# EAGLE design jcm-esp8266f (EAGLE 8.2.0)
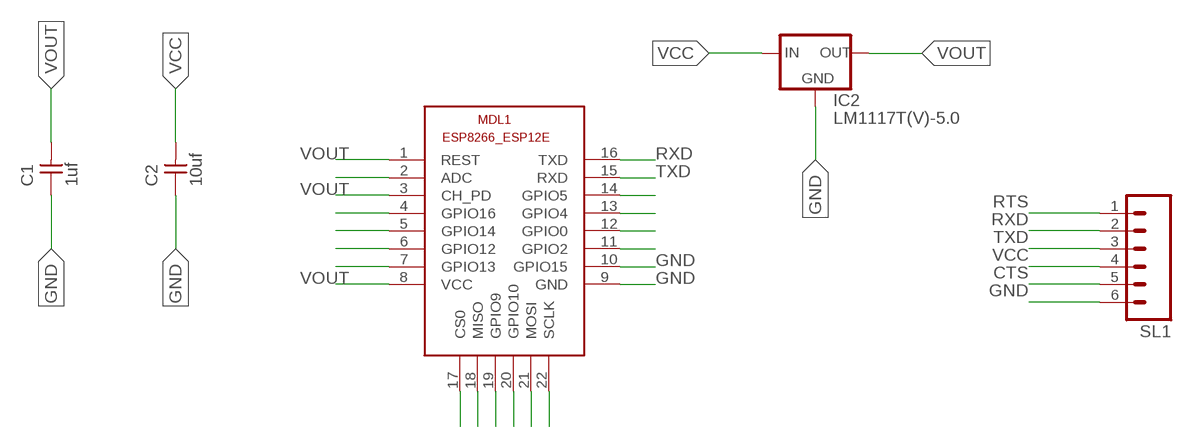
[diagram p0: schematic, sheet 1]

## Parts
C1  1uf  UNPOLARIZED_CAPACITOR1206  [1206]
C2  10uf  UNPOLARIZED_CAPACITOR1206  [1206]
IC2  LM1117T(V)-5.0  [TO220V]
MDL1  ESP8266-12EESP8266-ESP12E  [ESP8266-ESP12E]
SL1  M06  [06P]

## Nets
CTS: SL1.5
GND: C1.1 C2.1 IC2.1(GND) MDL1.9(GND) MDL1.10(GPIO15) SL1.6
N$9: MDL1.14(GPIO5)
N$10: MDL1.13(GPIO4)
N$11: MDL1.12(GPIO0)
N$12: MDL1.11(GPIO2)
N$15: MDL1.22(SCLK)
N$16: MDL1.21(MOSI)
N$17: MDL1.20(GPIO10)
N$18: MDL1.19(GPIO9)
N$19: MDL1.18(MISO)
N$20: MDL1.17(CS0)
N$22: MDL1.7(GPIO13)
N$23: MDL1.6(GPIO12)
N$24: MDL1.5(GPIO14)
N$25: MDL1.4(GPIO16)
N$27: MDL1.2(ADC)
RTS: SL1.1
RXD: MDL1.16(TXD) SL1.2
TXD: MDL1.15(RXD) SL1.3
VCC: C2.2 IC2.3(IN) SL1.4
VOUT: C1.2 IC2.2(OUT) MDL1.1(REST) MDL1.3(CH_PD) MDL1.8(VCC)

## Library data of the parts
C1 C2 = FAB_Hello:UNPOLARIZED_CAPACITOR: unpolarized_capacitor
IC2 = voltage_regulator:LM1117?-*: 800mA Low-Dropout Linear Regulator Source: http://ww1.microchip.com/downloads/en/DeviceDoc/39760d.pdf; MF: Texas Instruments; MPN: LM1117T-5.0; OC_FARNELL: 1215183; OC_NEWARK: 41K3491
MDL1 = ESP8266-ESP12E:ESP8266-12E: ESP8266-12E with additional I/O and GPIO04/05 corrected The author cannot warrant that this library is free from error or will meet your specific requirements. Created by PuceBaboon.com. Komagane, Nagano, JAPAN
SL1 = con-amp-quick:M06: AMP QUICK CONNECTOR; OC_FARNELL: unknown; OC_NEWARK: unknown

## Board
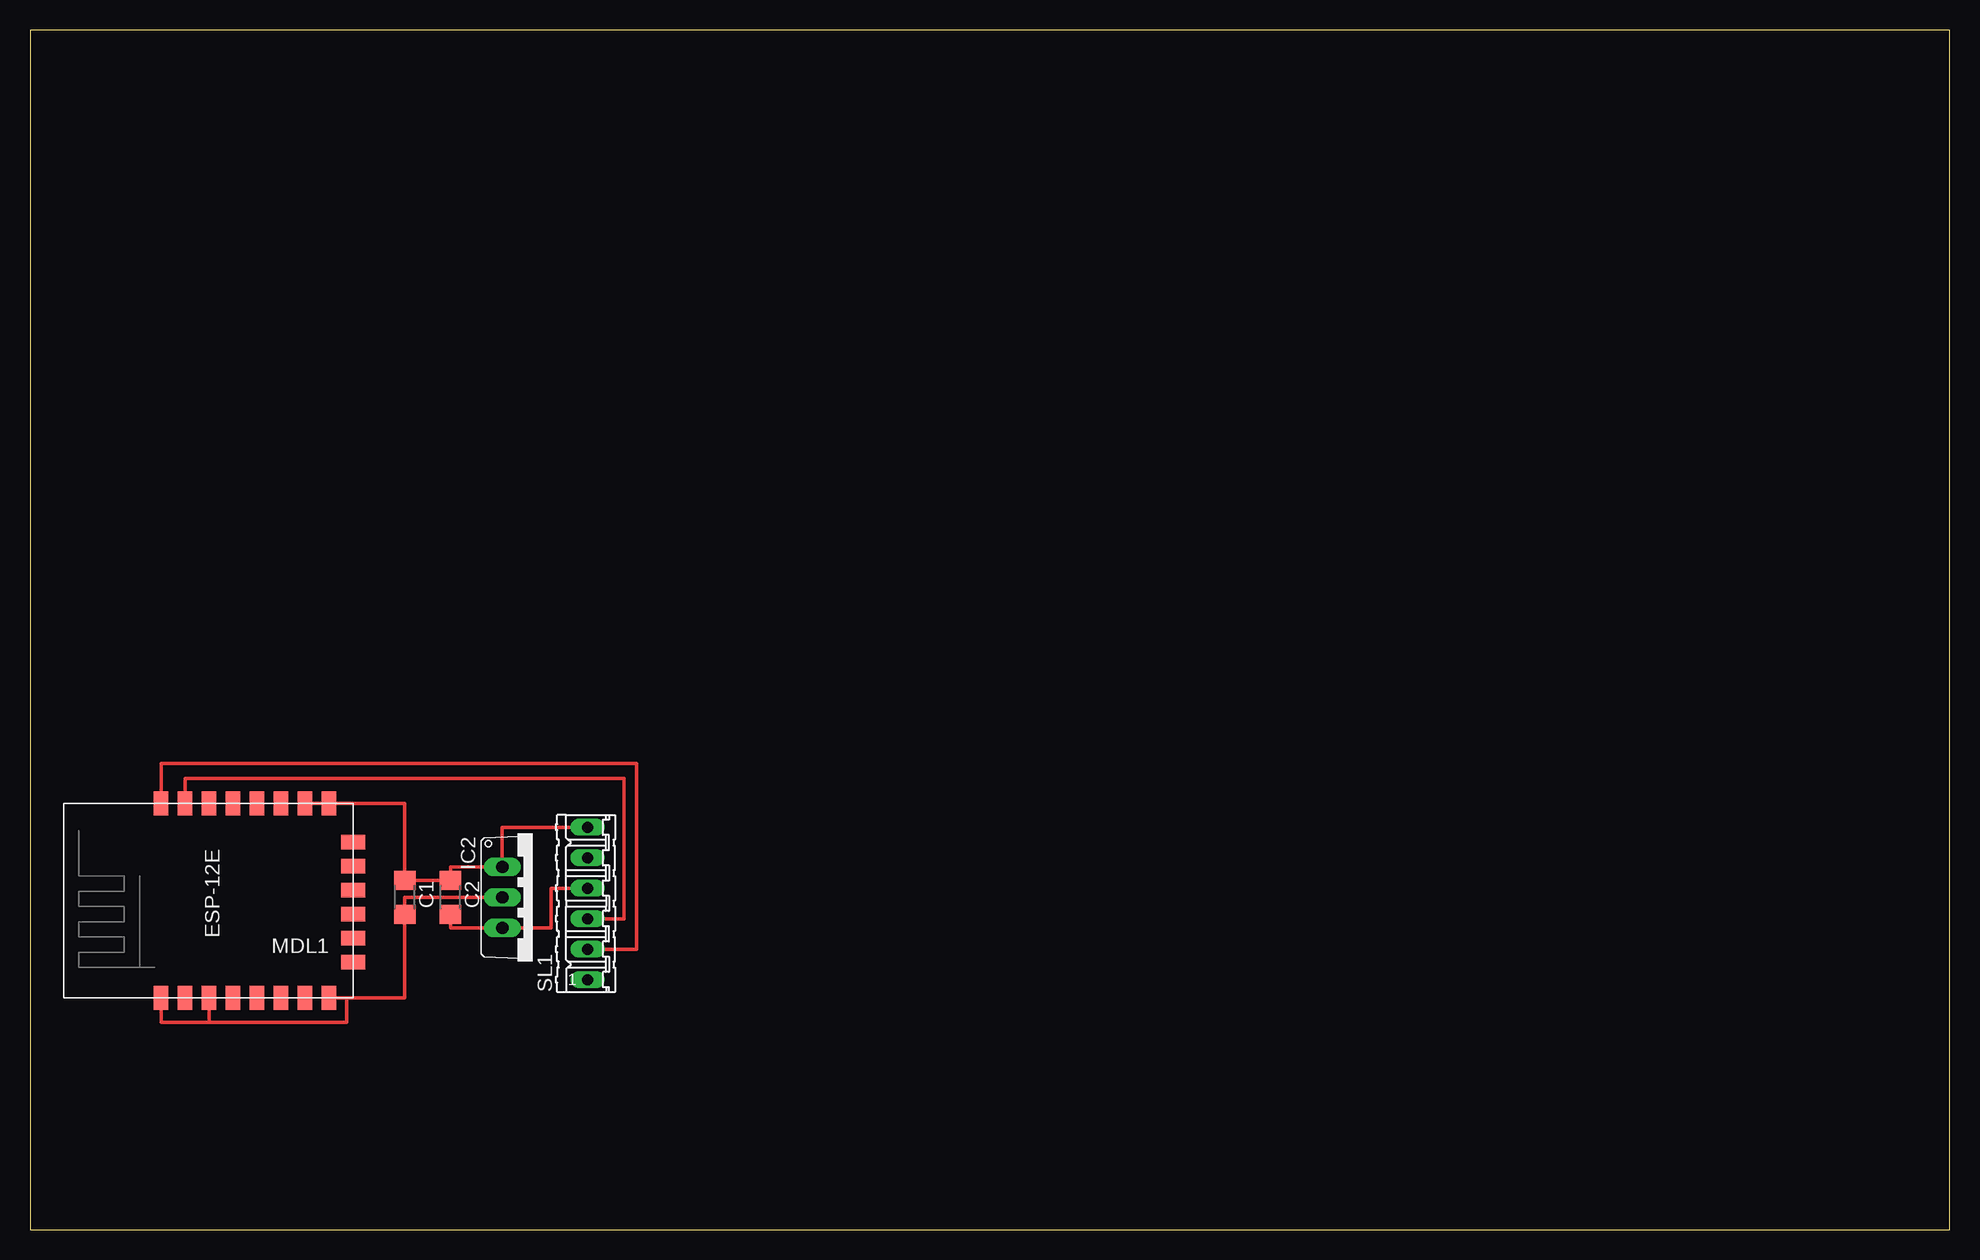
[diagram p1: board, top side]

Size 160 x 100 mm. Coordinates in mm from the lower left corner, seen from the top.
Outline: 0,0 160,0 160,100 0,100 0,0
Copper layers (1*16): Top 0.035mm / dielectric 1.5mm / Bottom 0.035mm
Design rules "default *": minimum track width 10mil, minimum drill 24mil, track to track 15mil, track to pad 15mil, pad to pad 15mil, via to via 15mil, smd to smd 15mil, copper to edge 40mil, drill to drill 8mil, minimum pad ring 10mil, minimum via ring 8mil, stop-mask expansion 4mil, vias tented up to drill 0mil, thermal gap 10mil

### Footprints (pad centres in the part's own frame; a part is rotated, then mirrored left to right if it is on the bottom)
1206 = smd 1.6 x 1.803: 1 -1.422,0; 2 1.422,0
TO220V = drill 1.016 long: 1 -2.54,-2.54; 2 0,-2.54; 3 2.54,-2.54
ESP8266-ESP12E = smd 2 x 1.2: 1 -7.62,5.84; 2 -7.62,3.84; 3 -7.62,1.84; 4 -7.62,-0.16; 5 -7.62,-2.16; 6 -7.62,-4.16; 7 -7.62,-6.16; 8 -7.62,-8.16; 9 8.58,-8.16; 10 8.58,-6.16; 11 8.58,-4.16; 12 8.58,-2.16; 13 8.58,-0.16; 14 8.58,1.84; 15 8.58,3.84; 16 8.58,5.84 | smd 1.2 x 2: 17 -4.62,-10.16; 18 -2.62,-10.16; 19 -0.62,-10.16; 20 1.38,-10.16; 21 3.38,-10.16; 22 5.38,-10.16
06P = drill 0.914 long: 1 -6.35,0; 2 -3.81,0; 3 -1.27,0; 4 1.27,0; 5 3.81,0; 6 6.35,0

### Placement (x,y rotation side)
C1  31.24,27.69 270 top
C2  35.05,27.69 270 top
IC2  41.91,27.69 270 top
MDL1  16.76,26.92 90 top
SL1  46.48,27.18 90 top

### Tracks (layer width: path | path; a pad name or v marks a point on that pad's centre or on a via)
GND
  Top 0.305: SL1.6 39.37,33.53 IC2.1 35.05,30.23 C2.1 C1.1 31.24,35.5 MDL1.9 MDL1.10
RXD
  Top 0.305: SL1.2 50.55,23.37 50.55,38.86 10.92,38.86 MDL1.16
TXD
  Top 0.305: SL1.3 49.53,25.91 49.53,37.59 12.95,37.59 12.95,35.05 12.92,35.05 MDL1.15
VCC
  Top 0.305: SL1.4 43.43,28.45 43.43,25.15 IC2.3 35.05,25.15 C2.2
VOUT
  Top 0.305: IC2.2 31.24,27.69 C1.2 31.24,19.3 26.42,19.3 | 26.42,19.3 MDL1.8 | MDL1.1 10.92,17.27 14.99,17.27 | 14.99,17.27 26.42,17.27 26.42,19.3 | MDL1.3 14.92,17.27 14.99,17.27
